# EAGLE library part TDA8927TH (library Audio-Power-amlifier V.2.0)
Power stage 2 ´ 80 W class-D audio amplifier
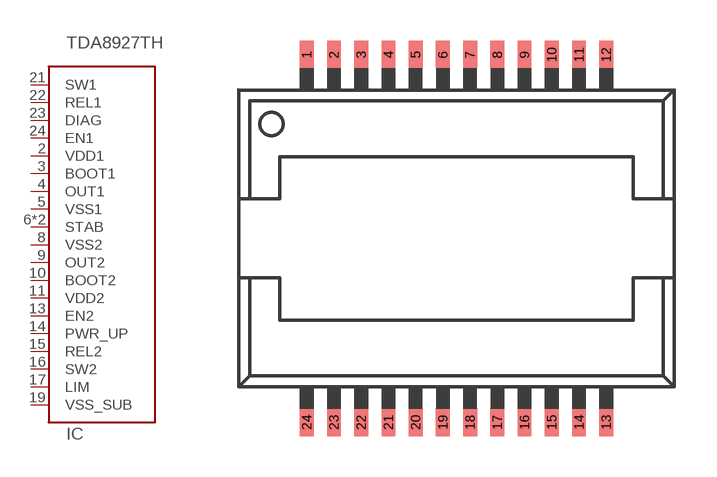
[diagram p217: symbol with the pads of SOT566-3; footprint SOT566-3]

Designator prefix IC

## TDA8927TH  [SOT566-3]
2  VDD1  pwr
3  BOOT1
4  OUT1  out
5  VSS1  pwr
6  STAB
7  STAB
8  VSS2  pwr
9  OUT2  out
10  BOOT2
11  VDD2  pwr
13  EN2  in
14  PWR_UP  in
15  REL2  out
16  SW2  in
17  LIM
19  VSS_SUB  pwr
21  SW1  in
22  REL1  out
23  DIAG  out
24  EN1  in

## Footprint SOT566-3 (pad centres in mm)
smd 0.508 x 1.016: 1 -5.5,6.75; 2 -4.5,6.75; 3 -3.5,6.75; 4 -2.5,6.75; 5 -1.5,6.75; 6 -0.5,6.75; 7 0.5,6.75; 8 1.5,6.75; 9 2.5,6.75; 10 3.5,6.75; 11 4.5,6.75; 12 5.5,6.75; 13 5.5,-6.75; 14 4.5,-6.75; 15 3.5,-6.75; 16 2.5,-6.75; 17 1.5,-6.75; 18 0.5,-6.75; 19 -0.5,-6.75; 20 -1.5,-6.75; 21 -2.5,-6.75; 22 -3.5,-6.75; 23 -4.5,-6.75; 24 -5.5,-6.75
